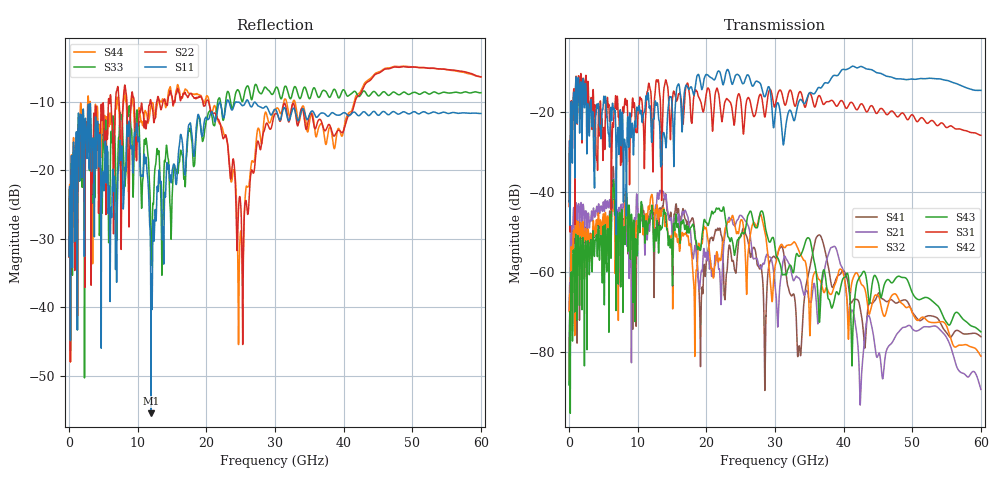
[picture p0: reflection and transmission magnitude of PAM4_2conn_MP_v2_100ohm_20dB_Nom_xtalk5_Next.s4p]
! Info: Touchstone file created by Circ.  Input file=FAB50GbE_2conn_Midplane_Examax_Topo2_v2_100ohm_20dB_Nom.circ
# Hz S RI R 50
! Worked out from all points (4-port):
!   6000 points, 10 MHz to 60 GHz, reference 50 ohm
!   strongest paths, dB at 10 MHz, 15.01 GHz, 30.01 GHz, 45.01 GHz, 60 GHz:
!     S42: -42.6, -18.4, -20.8, -10.2, -14.6
!     S31: -43.7, -17.6, -18.5, -20.0, -25.8
!     S43: -88.4, -56.1, -53.9, -62.5, -75.1
!     S32: -70.0, -54.4, -58.7, -66.0, -81.2
!     S21: -69.6, -50.5, -63.3, -81.0, -89.5
!     S41: -88.2, -49.5, -56.4, -65.6, -76.3
!   lowest |S11| = -55.5 dB at 11.94 GHz (marker M1), VSWR 1.00, Z = 50.1 + j0.102 ohm
!   |S11| at or under -10 dB: start of sweep to 22.97 GHz; 23.3 GHz to 25.75 GHz (2.447 GHz wide, 9.98 % of centre); 26.15 GHz to end of sweep
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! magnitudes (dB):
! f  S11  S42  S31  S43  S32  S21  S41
! 10 MHz  -32.5  -42.6  -43.7  -88.4  -70.0  -69.6  -88.2
! 1.54 GHz  -21.4  -25.3  -20.0  -64.8  -63.2  -51.1  -60.6
! 11.94 GHz  -55.5  -23.3  -15.5  -45.2  -41.1  -46.0  -45.8
! 24.87 GHz  -10.1  -11.1  -15.9  -51.6  -48.3  -45.9  -51.3
! 33.53 GHz  -12.5  -17.2  -15.1  -56.1  -55.0  -61.6  -78.6
! 36.39 GHz  -12.0  -13.8  -15.9  -70.3  -61.9  -70.2  -50.8
! 60 GHz  -11.7  -14.6  -25.8  -75.1  -81.2  -89.5  -76.3
